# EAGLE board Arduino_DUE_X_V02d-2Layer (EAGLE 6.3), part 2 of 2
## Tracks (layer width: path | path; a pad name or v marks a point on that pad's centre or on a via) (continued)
PIN41  (via drill 0.41) (continued)
  Top 0.203: U1.67 39.49,19.79 39.62,19.91 53.24,19.91 54.15,20.83 55.68,20.83 56.49,20.02 58.12,20.02 v58.37,20.27 | v61.47,20.62 61.67,20.42 62.89,20.42 63.2,20.73 65.94,20.73 68.28,23.06 71.83,23.06 74.47,25.7 81.79,25.7 81.99,25.91 91.03,25.91 92.76,24.18 95.3,24.18 XIO.22
  Bottom 0.203: v58.37,20.27 58.73,20.62 v61.47,20.62
PIN42  (via drill 0.41)
  Top 0.203: v58.32,19.2 58.01,19.2 57.61,19.61 56.29,19.61 55.47,20.42 54.36,20.42 53.44,19.51 42.06,19.51 41.05,18.49 39.52,18.49 39.22,18.19 39.22,17.98 39.02,17.79 U1.71 | v61.47,19.61 61.87,20.02 63.09,20.02 63.4,20.32 66.14,20.32 68.38,22.55 71.93,22.55 74.68,25.3 82.09,25.3 82.3,25.5 90.83,25.5 93.17,23.16 93.67,23.16 XIO.23
  Bottom 0.203: v58.32,19.2 58.83,19.61 v61.47,19.61
PIN43  (via drill 0.41)
  Top 0.203: v39.93,17.78 39.42,17.27 38,17.27 U1.72 | v40.03,28.65 40.44,28.14 42.67,28.14 43.38,28.85 49.48,28.85 49.68,28.65 55.58,28.65 v55.68,28.75 | v57.4,41.35 58.32,42.27 60.55,42.27 61.37,43.08 62.08,43.08 63.7,41.45 65.84,41.45 66.04,41.25 75.39,41.25 76,41.86 79.65,41.86 80.06,42.27 82.09,42.27 82.6,42.77 84.94,42.77 v85.34,42.37 | XIO.24 97.74,24.08 97.74,33.83 97.23,34.34 90.73,34.34 90.53,34.54 89.31,34.54 89.1,34.34 87.88,34.34 86.56,35.66 86.56,36.68 v85.95,37.29
  Bottom 0.203: v39.93,17.78 39.93,18.19 43.18,21.44 43.18,27.03 42.06,28.14 41.15,28.14 40.64,28.65 v40.03,28.65 | v57.4,41.35 57.1,41.05 57.1,36.37 59.64,33.83 59.64,30.38 58.42,29.16 56.08,29.16 v55.68,28.75 | v85.34,42.37 85.45,42.27 85.45,41.25 85.14,40.95 85.14,38.1 v85.95,37.29
PIN44  (via drill 0.41)
  Top 0.203: U1.101 54.15,16.05 54.46,16.36 54.46,17.27 53.34,18.39 v52.83,18.39 | v63.4,16.66 63.7,16.36 69.29,16.36 75.59,10.06 85.55,10.06 89.41,13.92 89.41,16.76 92.96,20.32 XIO.25
  Bottom 0.203: v52.83,18.39 53.24,18.39 54.46,17.17 54.46,16.36 54.15,16.05 54.15,13.51 55.68,11.99 57.91,11.99 58.93,13.01 60.76,13.01 61.77,14.02 61.77,15.75 62.69,16.66 v63.4,16.66
PIN45  (via drill 0.41)
  Top 0.203: v53.75,16.76 53.75,16.26 53.65,16.15 U1.100 | XIO.26 95.3,19.1 92.86,19.1 89.92,16.15 89.92,13.72 85.85,9.65 75.39,9.65 69.09,15.95 62.18,15.95 59.33,13.11 v59.33,12.19
  Bottom 0.203: v59.33,12.19 58.62,11.48 55.58,11.48 53.75,13.31 v53.75,16.76
PIN46  (via drill 0.41)
  Top 0.203: U1.99 53.15,16.05 53.03,16.15 53.03,17.12 v51.77,18.39 | v62.59,15.24 62.89,15.54 68.89,15.54 75.18,9.25 86.06,9.25 90.42,13.61 90.42,15.44 92.76,17.78 XIO.27
  Bottom 0.203: v51.77,18.39 53.03,17.12 53.03,15.85 53.34,15.54 53.34,13.11 55.47,10.97 59.64,10.97 62.59,13.92 v62.59,15.24
PIN47  (via drill 0.41)
  Top 0.203: v52.22,16.87 52.63,16.46 52.63,15.24 U1.98 | XIO.28 95.2,16.46 93.37,16.46 90.93,14.02 90.93,13.41 84.84,7.32 79.86,7.32 78.33,8.84 74.98,8.84 68.68,15.14 64.52,15.14 v64.21,14.83
  Bottom 0.203: v52.22,16.87 52.22,15.95 52.93,15.24 52.93,12.9 55.37,10.46 59.84,10.46 v64.21,14.83
PIN48  (via drill 0.41)
  Top 0.203: XIO.29 93.37,15.24 85.04,6.91 79.65,6.91 78.13,8.43 74.78,8.43 68.78,14.43 v65.23,14.43 | v50.7,18.39 51.51,17.58 51.51,16.56 52.15,15.93 U1.97
  Bottom 0.203: v50.7,18.39 51.51,17.58 51.51,15.95 52.53,14.94 52.53,12.7 55.27,9.96 60.76,9.96 v65.23,14.43
PIN49  (via drill 0.41)
  Top 0.203: XIO.30 95.3,14.02 92.76,14.02 85.24,6.5 79.45,6.5 77.93,8.03 74.57,8.03 68.89,13.72 61.98,13.72 58.83,10.57 53.65,10.57 v52.93,11.28 | v51.82,13.61 51.61,13.82 51.61,15.04 U1.96
  Bottom 0.203: v51.82,13.61 51.82,12.39 v52.93,11.28
PIN50  (via drill 0.41)
  Top 0.203: U1.95 51.13,16.13 51.04,16.22 51.04,16.73 v50.8,16.97 | v51.92,11.28 53.03,10.16 59.03,10.16 62.18,13.31 68.68,13.31 74.37,7.62 77.72,7.62 79.25,6.1 85.45,6.1 91.24,11.89 92.05,11.89 92.86,12.7 XIO.31
  Bottom 0.203: v50.8,16.97 50.8,16.46 51.1,16.15 51.1,12.09 v51.92,11.28
PIN51  (via drill 0.41)
  Top 0.203: XIO.32 95.3,11.48 91.44,11.48 85.65,5.69 79.05,5.69 77.52,7.21 74.17,7.21 68.48,12.9 62.38,12.9 59.23,9.75 52.43,9.75 v51.92,10.26 | 50.6,15.23 U1.94 50.65,16 50.09,16.56 50.09,17.88 v49.58,18.39
  Bottom 0.203: v49.58,18.39 50.09,17.88 50.09,15.85 50.7,15.24 50.7,11.48 v51.92,10.26
PWM2  (via drill 0.41)
  Top 0.203: U1.144 59.54,34.75 60.86,34.75 v61.06,34.54
  Bottom 0.203: v61.06,34.54 60.15,34.54 57.91,36.78 57.91,39.62 58.83,40.54 58.83,48.97 58.42,49.38 PWML.3 58.42,50.9
PWM3  (via drill 0.41)
  Top 0.203: v56.49,31.8 56.69,32 58.32,32 58.62,32.31 59.54,32.31 U1.139
  Bottom 0.203: PWML.4 55.88,49.38 55.58,49.07 55.58,48.06 55.88,47.75 55.88,36.68 55.58,36.37 55.58,33.43 56.49,32.51 v56.49,31.8
PWM5  (via drill 0.41)
  Top 0.203: U1.136 58.62,30.79 58.22,31.19 57.51,31.19 57,30.68 54.76,30.68 54.46,30.38 51.41,30.38 v51.1,30.68
  Bottom 0.203: v51.1,30.68 51.1,34.85 51.61,35.36 51.61,37.39 52.22,37.9 52.22,38.71 53.14,39.62 53.14,46.43 50.8,48.77 PWML.6
PWM6  (via drill 0.41)
  Top 0.203: v57.81,30.48 58.32,30.48 58.52,30.28 59.54,30.28 U1.135 | PWML.7 48.26,49.51 48.59,49.17 55.88,49.17 v56.39,48.67
  Bottom 0.203: v57.81,30.48 57.81,31.9 55.98,33.73 55.98,35.66 56.29,35.97 56.29,48.56 v56.39,48.67
PWM7  (via drill 0.41)
  Top 0.203: U1.134 59.66,29.79 59.64,29.77 57.51,29.77 57,30.28 54.97,30.28 54.66,29.97 50.49,29.97 50.39,30.07 45.41,30.07 v45.11,30.38
  Bottom 0.203: v45.11,30.38 45.11,33.53 44.6,34.04 44.6,37.59 44.5,37.69 44.5,38.51 44.81,38.81 44.81,45.41 45.11,45.72 45.11,48.16 45.72,48.77 PWML.8
PWM8  (via drill 0.41)
  Top 0.203: v42.57,29.77 42.67,29.67 50.09,29.67 50.29,29.46 54.76,29.46 55.17,29.87 56.79,29.87 57.4,29.26 59.54,29.26 U1.133
  Bottom 0.203: PWMH.1 41.66,48.77 40.84,47.95 40.84,38.41 41.76,37.49 41.76,34.75 42.47,34.04 42.47,29.87 v42.57,29.77
PWM9  (via drill 0.41)
  Top 0.203: U1.132 59.43,28.79 59.33,28.78 57.28,28.78 56.59,29.46 55.37,29.46 54.97,29.06 49.99,29.06 49.78,29.26 43.18,29.26 42.77,28.85 v41.45,28.85
  Bottom 0.203: PWMH.2 39.12,49.07 40.44,47.75 40.44,38.2 40.95,37.69 40.95,34.34 42.06,33.22 42.06,30.28 41.45,29.67 v41.45,28.85
PWM11  (via drill 0.41)
  Top 0.203: v48.06,38.51 48.06,37.9 48.16,37.8 48.16,36.98 U1.20 | v39.32,45.52 39.73,45.52 39.83,45.41 44.7,45.41 45.31,46.02 46.43,46.02 46.74,46.33 47.55,46.33 47.95,45.92 47.95,45.41 v48.46,44.91
  Bottom 0.203: v48.46,44.91 47.85,44.3 47.85,39.22 48.06,39.01 v48.06,38.51 | PWMH.4 34.04,49.07 35.15,47.95 37.19,47.95 39.32,45.82 v39.32,45.52
PWM12  (via drill 0.41)
  Top 0.203: U1.21 47.65,35.46 v47.95,35.15 | v47.24,49.28 44.2,49.28 43.99,49.48 42.47,49.48 42.27,49.28 31.8,49.28 31.5,49.58 PWMH.5
  Bottom 0.203: v47.95,35.15 47.75,35.36 47.75,37.69 47.35,38.1 47.35,39.01 47.45,39.12 47.45,44.91 48.36,45.82 48.36,48.16 v47.24,49.28
PWM13  (via drill 0.41)
  Top 0.203: 21.34,28.25 IC1.3 | U1.68 35.87,19.3 35.78,19.29 31.27,19.29 v30.79,18.8
  Top 0.305: v22.96,28.25 21.34,28.25
  Bottom 0.203: PWMH.6 26.92,48.77 26.92,34.19 22.96,30.23 v22.96,28.25 23.47,28.25 27.33,24.38 27.43,24.38 28.75,23.06 28.75,20.83 v30.79,18.8
RD+
  Top 0.254: IC6.29 17.94,23.41 16.26,25.09 R20.1
RD-
  Top 0.254: IC6.30 17.44,23 16.46,23.98 15.04,23.98 14.98,24.02 R19.1
RESET2  (via drill 0.41)
  Top 0.254: ICSP1.5 26.01,17.27 26.01,18.29 26.21,18.49 26.21,19.33 D2.A | R13.1 22.55,23.84 v22.55,22.45 21.95,22.45 21.54,22.05 21.54,21.54 21.26,21.26 IC6.24
  Bottom 0.254: v22.55,22.45 23.37,23.27 24.38,23.27 24.89,22.76 24.89,20.73 24.49,20.32 24.49,18.85 25.91,17.37 | 25.96,17.32 ICSP1.5
  Bottom 0.305: 25.91,17.37 25.96,17.32
RESET_CMD
  Top 0.254: IC6.22 21.97,20.26 R23.1
RX  (via drill 0.41)
  Top 0.203: U1.27 44.65,35.01 45.31,34.34 v48.67,34.34 | v49.07,47.85 49.58,48.36 52.02,48.36 52.73,47.65 53.14,47.65 54.05,48.56 55.47,48.56 56.08,47.95 57.71,47.95 58.52,48.77 62.99,48.77 63.5,49.28 PWML.1 63.5,52 62.92,52.58 18.64,52.58 17.68,51.61 17.68,48.46 17.41,48.2 12.58,48.2 v12.2,48.58
  Top 0.254: IC10.4 13.95,15.45 v13.38,16.4
  Bottom 0.203: v48.67,34.34 48.67,35.76 48.77,35.87 48.77,38.91 48.26,39.42 48.26,43.69 49.28,44.7 49.28,46.13 49.07,46.33 v49.07,47.85 | v13.38,16.4 13.38,16.83 14.22,17.68 14.22,20.02 16.15,21.95 16.15,23.67 13.11,26.72 13.11,40.95 13.82,41.66 13.82,43.89 13.11,44.6 13.11,47.04 12.19,47.95 v12.19,48.57 v12.2,48.58
RXD0  (via drill 0.41)
  Top 0.203: COMMUNICATION.2 71.12,49.07 70.81,48.77 69.39,48.77 67.97,47.35 65.13,47.35 64.52,47.95 58.93,47.95 58.12,47.14 55.68,47.14 55.07,47.75 54.46,47.75 53.54,46.84 52.32,46.84 51.82,47.35 50.8,47.35 v50.09,46.63 | U1.18 49.15,37.62 49.48,37.95 v49.48,38.41
  Bottom 0.203: v50.09,46.63 50.09,45.52 49.78,45.21 49.78,44.6 48.67,43.48 48.67,39.62 49.48,38.81 v49.48,38.41
RXD1  (via drill 0.41)
  Top 0.203: v58.83,38.71 56.07,38.71 55.68,38.32 55.68,36.98 U1.5 | COMMUNICATION.4 76.2,48.36 75.79,47.95 70.92,47.95 v70.61,47.65
  Bottom 0.203: v58.83,38.71 58.83,39.93 59.23,40.34 59.23,47.14 60.25,48.16 70.1,48.16 v70.61,47.65
RXD2  (via drill 0.41)
  Top 0.203: U1.3 56.65,37.75 56.79,37.9 57.81,37.9 58.12,37.59 59.44,37.59 60.25,38.41 v60.66,38.41 | COMMUNICATION.6 81.28,48.46 80.87,48.06 79.96,48.06 79.45,47.55 77.42,47.55 77.01,47.14 72.95,47.14 v72.64,46.84
  Bottom 0.203: v60.66,38.41 61.37,39.12 61.37,39.83 60.45,40.74 60.45,46.53 60.86,46.94 66.34,46.94 67.16,46.13 71.93,46.13 v72.64,46.84
RXL  (via drill 0.41)
  Top 0.203: 55.17,15.23 U1.103 55.15,14.1 v54.86,13.92 | v32.31,15.75 33.73,15.75 34.54,16.56 35.26,16.56 35.56,16.26 40.34,16.26 41.45,17.37 43.38,17.37 44.4,18.39 v44.91,18.39
  Top 0.508: RX.C 7.92,33.33 6.81,32.21 v6.81,29.77
  Bottom 0.203: v54.86,13.92 54.86,17.37 53.14,19.1 48.06,19.1 47.75,18.8 47.75,17.88 47.24,17.37 45.92,17.37 v44.91,18.39 | v32.31,15.75 29.67,13.11 29.67,11.89 28.65,10.87 23.77,10.87 22.15,9.25 17.17,9.25 14.02,12.39 5.89,12.39 3.56,14.73 3.56,16.97 6.81,20.22 v6.81,29.77
RXL-U2
  Top 0.254: IC6.10 16.94,16.24 15.7,15 15.7,13.6 15,12.9 15,12.87 14.33,12.19 7.62,12.19 6.6,13.21 6.6,14.02 5.38,15.24 5.38,16.49 RX1.C
SCK2  (via drill 0.41)
  Top 0.254: IC6.15 19.44,16.08 v18.9,15.54
  Bottom 0.203: v18.9,15.54 18.9,16.87 19.61,17.58 21.13,17.58 22.76,15.95 24.74,15.95 ICSP1.3
SCL0-3  (via drill 0.41)
  Top 0.203: v57.71,28.04 57.25,27.64 54.76,27.64 54.56,27.84 47.09,27.84 v46.99,27.74 | v46.99,18.39 46.99,17.42 46.84,17.27 46.84,16.46 47.14,16.15 U1.87 | v85.95,38.41 85.34,39.01 81.48,39.01 81.42,38.95 80.5,38.95 79.5,37.95 | 79.5,37.95 78.23,36.68 68.89,36.68 67.16,38.41 64.92,38.41 63.09,36.58 63.09,35.36 62.48,34.75 v62.48,33.43 | RN5.7 80.77,36.68 79.5,37.95
  Bottom 0.203: v62.48,33.43 62.08,33.43 61.37,32.72 61.09,32.72 60.55,32.18 60.55,30.07 58.52,28.04 v57.71,28.04 | v46.99,18.39 46.94,24.23 46.63,24.54 46.63,27.38 v46.99,27.74
  Bottom 0.254: COMMUNICATION.8 86.26,50.7 86.26,42.16 85.95,41.86 v85.95,38.41
SCL1  (via drill 0.41)
  Top 0.203: 38,18.29 U1.70 37.19,18.29 37.08,18.39 34.95,18.39 34.34,17.78 33.63,17.78 33.53,17.88 v32.41,17.88 | PWMH.10 18.8,50.29 19.71,49.38 22.55,49.38 23.27,48.67 26.31,48.67 27.03,49.38 29.77,49.38 v29.87,49.48
  Bottom 0.203: v29.87,49.48 29.87,46.94 29.46,46.53 29.46,42.06 28.85,41.45 28.85,32.26 29.87,31.24 29.87,24.89 31.8,22.96 31.8,20.32 32.31,19.81 32.31,17.98 v32.41,17.88
SDA0-3  (via drill 0.41)
  Top 0.203: U1.86 46.63,15.34 | 46.63,15.34 46.69,15.24 | 46.63,15.34 46.63,16.01 46.38,16.26 46.38,17.98 v45.97,18.39 | v55.58,23.98 55.37,23.67 52.73,23.67 51.82,22.76 46.63,22.76 46.33,23.06 v45.97,23.06 | v79.45,36.47 79.25,36.47 78.94,36.17 71.22,36.17 v69.6,34.54
  Top 0.254: RN5.8 80.04,35.88 v79.45,36.47
  Bottom 0.203: v45.97,18.39 v45.97,23.06 | v55.58,23.98 55.68,25.2 57.3,26.82 58.52,26.82 61.77,30.07 61.77,31.29 62.79,32.31 66.95,32.31 69.09,34.54 v69.6,34.54
  Bottom 0.254: COMMUNICATION.7 83.82,43.69 82.91,42.77 82.91,40.44 82.7,40.23 82.7,38.2 81.99,37.49 80.47,37.49 v79.45,36.47
SDA1  (via drill 0.41)
  Top 0.203: v52.93,48.46 52.63,48.77 48.77,48.77 48.56,48.56 46.94,48.56 46.63,48.87 44.4,48.87 43.38,47.85 43.08,47.85 42.47,48.46 38.51,48.46 38,47.95 28.75,47.95 28.55,48.16 27.74,48.16 27.03,47.45 20.83,47.45 v20.02,48.26 | U1.9 53.65,36.78 53.65,35.56 v52.83,34.75
  Bottom 0.203: v52.93,48.46 53.54,47.85 53.54,39.42 52.63,38.51 52.63,35.56 52.83,35.36 v52.83,34.75 | v20.02,48.26 20.02,48.97 21.03,49.99 21.03,50.6 21.13,50.7 PWMH.9
SPCK  (via drill 0.41)
  Top 0.203: v72.54,28.85 69.7,28.85 69.19,28.35 67.67,28.35 66.75,29.26 65.33,29.26 64.72,28.65 64.41,28.65 SPI.3 | U1.110 60.66,17.79 62.48,19.61 63.3,19.61 63.6,19.91 66.34,19.91 68.48,22.05 71.53,22.05 v71.73,21.84
  Bottom 0.203: v71.73,21.84 71.73,25.6 72.54,26.52 v72.54,28.85
SS0/PWM10  (via drill 0.41)
  Top 0.203: U1.102 54.66,15.24 54.66,15.95 54.86,16.15 54.86,17.48 53.65,18.69 53.65,19.1 | U1.111 59.54,18.29 59.03,18.29 58.73,17.98 57.35,17.98 57.15,18.19 56.13,18.19 55.78,18.54 55.78,19.51 55.27,20.02 54.56,20.02 53.65,19.1 | v46.33,48.16 44.3,48.16 43.59,47.45 42.88,47.45 42.27,48.06 41.45,48.06 40.95,47.55 39.01,47.55 v38.91,47.75 | 53.65,19.1 43.69,19.1 v43.38,18.8
  Bottom 0.203: v38.91,47.75 36.58,50.09 PWMH.3 | v46.33,48.16 46.74,47.75 46.74,46.94 45.92,46.13 45.92,45.31 45.62,45.01 45.62,38.81 45.92,38.51 45.92,37.8 45.01,36.98 45.01,34.44 45.82,33.63 45.82,29.67 44.81,28.65 44.81,20.22 v43.38,18.8
SS1/PWM4  (via drill 0.41)
  Top 0.203: v53.54,31.09 56.79,31.09 57.3,31.6 58.42,31.6 58.73,31.29 59.54,31.29 U1.137 | U1.112 58.96,18.79 58.65,18.49 57.61,18.49 57.1,18.9 v56.49,18.9
  Bottom 0.203: PWML.5 53.44,50.8 53.44,49.38 55.47,47.35 55.47,36.98 55.17,36.68 55.17,34.44 53.54,32.82 v53.54,31.09 53.54,22.35 56.49,19.41 v56.49,18.9
SW
  Top 0.406: 82.98,17.92 D4.P$1 | IC2.6 83.24,15.89 C42.2
  Top 0.61: C42.2 82.98,17.92
  Top 1.27: 82.21,20.79 L4.P$1
  Top 1.676: D4.P$1 82.21,20.79
  pour Top (isolate 0.406, no thermals): 85.55,24.28 82.8,24.28 80.57,22.15 80.57,17.48 80.98,17.17 81.69,17.17 82.09,16.76 82.09,14.43 83.52,14.43 83.52,20.32 85.55,22.35
TX  (via drill 0.41)
  Top 0.203: U1.2 57.15,36.02 56.69,35.55 56.69,35.11 v56.69,35.05 | v57.4,48.67 57.91,49.17 60.66,49.17 60.96,49.48 PWML.2
  Top 0.254: IC6.8 14.93,17.76 14.72,17.57 v14.73,16.85
  Bottom 0.203: v56.69,35.05 56.69,47.95 v57.4,48.67 | PWML.2 59.18,52.58 21.18,52.58 20.12,51.51 20.12,49.78 19.2,48.87 17.98,48.87 16.66,47.55 14.43,47.55 13.51,46.63 13.51,45.01 14.22,44.3 14.22,41.15 13.61,40.54 13.61,26.82 16.56,23.88 16.56,21.74 14.63,19.81 14.63,16.95 v14.73,16.85
TXD0  (via drill 0.41)
  Top 0.203: U1.17 49.65,35.39 v49.38,35.15 | v50.09,47.65 50.39,47.95 51.82,47.95 52.53,47.24 53.34,47.24 54.25,48.16 55.27,48.16 55.88,47.55 57.91,47.55 58.73,48.36 64.72,48.36 65.33,47.75 67.77,47.75 68.58,48.56 COMMUNICATION.1
  Bottom 0.203: v49.38,35.15 50.19,35.97 50.19,38.71 49.07,39.83 49.07,43.28 50.19,44.4 50.19,44.81 50.8,45.41 50.8,47.35 50.49,47.65 v50.09,47.65
TXD1  (via drill 0.41)
  Top 0.203: v54.46,35.05 55.12,35.61 55.12,36.83 55.12,36.84 U1.6 | COMMUNICATION.3 73.66,48.77 73.25,48.36 69.6,48.36 68.17,46.94 64.92,46.94 64.31,47.55 59.13,47.55 58.32,46.74 55.07,46.74 v54.76,47.04
  Bottom 0.203: v54.46,35.05 54.46,37.08 55.07,37.69 55.07,46.74 v54.76,47.04
TXD2  (via drill 0.41)
  Top 0.203: U1.4 56.15,38.06 56.39,38.3 58.01,38.3 58.32,38 59.23,38 v60.66,39.42 | COMMUNICATION.5 78.74,48.36 78.33,47.95 77.22,47.95 76.81,47.55 71.93,47.55 v71.63,47.24
  Bottom 0.203: v60.66,39.42 60.05,40.03 60.05,46.74 60.66,47.35 66.55,47.35 67.36,46.53 70.92,46.53 v71.63,47.24
TXL  (via drill 0.41)
  Top 0.203: v29.16,8.53 30.18,7.52 32,7.52 32.41,7.92 45.01,7.92 45.31,8.23 45.31,9.2 45.67,9.55 47.45,9.55 47.7,9.8 49.23,9.8 51.51,12.09 53.24,12.09 54.36,10.97 58.01,10.97 58.52,11.58 58.52,13.72 58.06,14.17 57.56,14.17 57.15,14.59 U1.107
  Top 0.508: TX.C 8.79,31.45 v8.03,30.68
  Bottom 0.203: v8.03,30.68 6.6,30.68 6.1,30.18 6.1,20.12 3.05,17.07 3.05,14.33 5.49,11.89 13.92,11.89 17.07,8.74 24.69,8.74 24.89,8.94 26.31,8.94 26.72,8.53 v29.16,8.53
TXL-U2
  Top 0.254: IC6.11 17.44,16.04 16.2,14.8 16.2,13.3 14.58,11.68 7.15,11.68 TX1.C
UOTGID  (via drill 0.41)
  Top 0.203: 48.11,26.57 48.46,26.92 54.25,26.92 54.46,26.72 58.01,26.72 58.58,27.29 U1.129
  Top 0.254: 48.11,26.57 43.43,26.57 42.72,27.28 41.1,27.28 40.64,26.82 v40.54,26.82 | v36.68,45.11 35.97,45.82 31.6,45.82 31.39,45.62 30.07,45.62 29.92,45.77 22.45,45.77 21.29,44.6 20.02,44.6 19.3,45.31 7.32,45.31 6.91,44.91 v5.79,44.91 | 4.06,37.44 4.37,37.44 | 4.37,37.44 5.36,37.44 v6.5,36.27 | USB1.4 4.39,37.45 arc45 4.37,37.44
  Top 0.305: Z5.2 5.67,44.79 v5.79,44.91
  Bottom 0.254: v40.54,26.82 39.52,26.82 37.59,28.75 37.59,34.54 36.78,35.36 36.78,45.01 v36.68,45.11 | v6.5,36.27 6.5,44.2 v5.79,44.91
UOTGVBOF  (via drill 0.41)
  Top 0.203: U1.128 59.49,26.77 58.78,26.77 58.32,26.31 54.15,26.31 54.05,26.42 48.67,26.42 48.36,26.11 42.77,26.11 v42.37,26.52 | v36.68,17.68 34.95,17.68 34.65,17.37 33.63,17.37 v33.33,17.07
  Top 0.305: v30.58,25.2 30.38,25.4 R3.1
  Bottom 0.203: v42.37,26.52 42.77,26.11 42.77,21.84 38.61,17.68 v36.68,17.68 | v33.33,17.07 33.33,17.68 33.12,17.88 33.12,19.71 32.31,20.52 32.31,23.47 v30.58,25.2
USBVCC  (via drill 0.41, 0.61)
  Top 0.305: R21.2 21.17,24.63 v21.84,25.3 | R2.2 19.16,43.12 18.57,43.61 C27.+
  Top 0.406: 13.71,43.8 C35.+
  Top 0.762: v15.34,28.25 14.83,28.25 14.63,28.45 14.38,28.45 T1.1
  Top 0.813: F1.1 14.63,41 14.63,43.79 | 14.63,43.79 14.43,43.79 14.04,43.8 C35.+ | 14.63,43.79 16.97,43.79 C27.+ | C27.+ 16.87,43.71 | C27.+ v16.97,41.66
  Bottom 0.406: v21.84,25.3 21.84,25.5 20.73,26.62 15.95,26.62 15.44,27.13 v15.34,28.25
  Bottom 0.813: v16.97,41.66 16.97,29.16 16.05,28.25 v15.34,28.25
USBVCCU2  (via drill 0.61)
  Top 0.254: IC6.31 16.94,22.59 16.46,23.06
  Top 0.305: 16.46,23.06 11.99,23.06 11.79,23.27 T2.1 | C28.1 3.5,31.05 F2.1
  Top 0.61: T2.1 10.74,23.88 10.74,24.21 v10.67,24.28 | v6.81,33.83 6.28,33.83 F2.1
  Bottom 0.61: v10.67,24.28 10.46,24.28 9.45,25.3 9.45,28.65 10.06,29.26 10.06,32 8.94,33.12 7.52,33.12 v6.81,33.83
VBG  (via drill 0.41)
  Top 0.203: v39.42,33.12 39.24,33.3 38.23,33.3 U1.40 | v38.41,37.54 35.92,37.54 35.51,37.13 31.45,37.13 31.29,37.29 29.55,37.29 C25.1 29.26,37.27 29.26,37.8 29.06,38 28.04,38 27.84,37.8 26.72,37.8 26.49,37.57 R7.2
  Bottom 0.203: v38.41,37.54 38.41,36.88 39.42,35.87 v39.42,33.12
VDDANA  (via drill 0.41)
  Top 0.203: 40.12,15.01 U1.73
  Top 0.305: v39.42,15.01 40.12,15.01
  Top 0.406: v39.42,15.01 39.05,15.38 C10.2 35.6,15.38 35.15,14.94 34.75,14.94 33.83,14.02 L1.2
  Top 0.508: C3.+ v39.42,9.55
  Bottom 0.406: v39.42,15.01 v39.42,9.55
VDDOUT  (via drill 0.41, 0.61)
  Top 0.203: 38,22.78 U1.61 38.2,22.76 | 35.36,30.48 C14.2 | 59.54,24.79 U1.124 | 35.36,25.4 C15.2 | 54.8,12.9 C16.2 | 36.37,43.79 L5.1 | C17.2 61.57,23.77 | 32.72,21.54 32.92,21.74 | C11.+ 32.56,22.3 32.51,22.35
  Top 0.254: 59.54,24.79 58.73,24.79 58.57,24.64 57.35,24.64 57.2,24.69 57.15,24.79 | C12.2 34.28,21.68 34.95,21.74 | U1.124 60.8,24.79 C17.2
  Top 0.279: U1.45 36.68,30.79 | U1.10 53.15,37.91 v53.44,38.2 | 55.32,16.56 55.65,16.29 U1.104 55.65,13.48 55.07,12.9 C16.2 | 35.46,25.3 35.46,25.4 C15.2 | 38,22.78 36.6,22.78 36.68,22.76
  Top 0.292: 36.49,25.29 U1.56 39.36,25.29
  Top 0.305: 35.36,30.48 v36.37,30.48 36.68,30.79 | 36.49,25.29 v36.37,25.3 35.46,25.3 | C13.2 53.44,39.32 v53.44,38.2 | 39.36,25.29 39.93,25.86 | 55.32,16.56 55.32,18.85 v55.07,19.2
  Top 0.406: 57.15,24.79 53.95,24.79 53.34,24.18 52.43,24.18 51.82,23.57 v51.1,23.57 51.16,23.52 51.16,24.69 50.34,25.5 42.16,25.5 41.81,25.86 39.93,25.86 | 36.68,22.76 v35.66,21.74
  Top 0.61: v35.36,43.59 35.41,43.79 36.37,43.79 36.37,43.84
  Top 0.813: v35.66,21.74 34.95,21.74 34.75,21.95 33.53,21.95 33.33,21.74 32.92,21.74 32.51,21.74 32.51,22.35
  Bottom 0.406: v53.44,38.2 53.44,36.37 53.65,36.17 53.65,34.24 52.73,33.43 52.73,26.21 52.83,26.11 52.83,25.3 v51.1,23.57 52.02,23.57 53.03,22.55 53.03,22.05 55.07,20.02 v55.07,19.2
  Bottom 0.61: v36.37,30.48 36.37,31.09 33.83,33.63 33.83,39.12 35.36,40.64 v35.36,43.59
  Bottom 0.813: v36.37,30.48 v36.37,25.3 36.37,22.45 v35.66,21.74
VDDOUTMI  (via drill 0.41)
  Top 0.203: C2.+ 29.11,39.77 29.06,39.83 | 31.29,39.42 L2.2
  Top 0.254: 35.39,32.78 35.36,32.78 35.36,32.72 C9.2
  Top 0.279: U1.41 35.39,32.78
  Top 0.305: 35.39,32.78 35.36,32.82 v35.36,33.58
  Top 0.406: v34.85,38.15 32.56,38.15 31.29,39.42
  Top 0.61: L2.2 30.13,39.42 C2.+
  Bottom 0.406: v35.36,33.58 35.36,37.64 v34.85,38.15
VDDPLL
  Top 0.203: 41.96,42.67 42.27,43.08 | 42.27,43.69 42.27,43.28 42.27,43.08 | 42.27,43.08 C33.+ | L5.2 38.61,43.79
  Top 0.279: U1.34 41.15,39.52
  Top 0.406: 41.15,39.52 41.96,40.34 | 41.96,40.34 41.96,42.67 | C32.2 41.96,40.34
  Top 0.61: 38.61,43.79 39.83,43.79 40.13,43.48 42.06,43.48 42.27,43.28
VIN  (via drill 0.41, 0.61)
  Top 0.305: v27.84,29.16 26.92,30.07 RN4.6
  Top 0.406: 84.96,15.67 v84.73,15.54
  Top 0.61: 84.96,15.67 C41.+ 87.21,15.02 87.21,14.06 87.07,13.92 R10.1 | v84.73,15.54 v84.73,14.33 83.92,13.51 IC2.5
  Top 1.016: v32,6.6 32.41,6.6 32.72,6.91 45.21,6.91 45.52,6.6 v45.72,6.6 | v32,6.6 32.11,6.6 | v32,6.6 27.23,6.6 24.22,3.59 PC1.+ 21,3.59 D5.P$1
  Bottom 0.305: v27.84,29.16 27.84,28.45 28.65,27.64 28.65,23.88 29.26,23.27 29.26,21.54 31.6,19.2 31.6,17.58 33.22,15.95 33.22,7.62 32.61,7.01 v32,6.6
  Bottom 0.61: v84.73,14.33 82.6,14.33 77.72,9.45 73.97,9.45 68.89,4.37 50.39,4.37 49.07,3.05 49.07,2.34 48.46,1.73 46.53,1.73 POWER.8
  Bottom 1.016: POWER.8 v45.72,6.6
  pour Top (no thermals): 87.78,16.56 85.04,16.56 84.12,15.65 84.12,13.61 85.04,13.61 85.24,13.82 85.24,14.43 85.55,14.73 87.68,14.73 87.88,14.94 87.88,16.46
  pour Bottom: 84.12,16.15 85.55,16.15 85.55,13.72 84.12,13.72
VIN+
  Top 1.016: X2.2 11.71,8.33 13.82,8.33 15.53,6.62 L6.2
VUCAP
  Top 0.254: IC6.27 18.94,23.87 C38.1
XIN
  Top 0.203: 36.47,41.76 Y1.1 | 36.47,41.76 36.27,41.35 | 36.47,41.76 36.58,41.86 Y1.1 | U1.36 40.15,37.58 39.37,38.35 35.87,38.35 34.91,39.31 34.91,40.2 | C22.1 34.91,40.2 | 34.91,40.2 35.55,40.2 35.97,40.64 35.97,41.15 Y1.1
XIN32
  Top 0.203: U1.48 38,29.26 37.29,29.26 36.98,29.57 33.12,29.57 32.31,30.38 31.24,30.38 | C24.1 31.01,30.48 | 31.01,30.48 31.24,30.38 | 31.24,30.38 Y2.P$2 31.01,30.48
XOUT
  Top 0.203: 39.57,39.47 38.41,39.47 38.41,39.62 Y1.3 38.41,39.42 | 39.57,39.47 39.58,39.47 40.23,40.13 40.23,40.84 C21.1 | U1.35 40.64,36.98 40.64,37.85 39.98,38.51 39.57,38.91 39.57,39.47
XOUT32
  Top 0.203: U1.49 38,28.79 38,28.8 37.03,28.8 36.68,29.16 33.53,29.16 32.31,27.94 31.7,27.94 | C23.1 31.22,27.84 | 31.22,27.84 31.7,27.94 | 31.7,27.94 Y2.P$1 31.22,27.84
XT1
  Top 0.254: C39.1 R9.1 | Y4.1 8.62,15.03 9.55,15.95 9.55,17.48 9.14,17.88 9.14,18.45 R9.1 | IC6.1 12.82,21.26 11.68,20.12 11.07,20.12 10.36,19.41 9.35,19.41 9.11,19.16 R9.1
XT2
  Top 0.254: 10.06,18.55 R9.2 C40.1 | Y4.3 10.7,18.16 C40.1 | IC6.2 13.24,20.76 12.09,19.61 11.38,19.61 11.04,19.27 C40.1
XUSB  (via drill 0.41)
  Top 0.254: USB1.1 4.42,39.4 arc45 4.47,39.4 | U1.39 36.62,33.78 v36.58,33.73 | v35.15,44.91 35.05,44.91 34.75,45.11 29.67,45.11 29.46,45.31 22.66,45.31 21.13,43.79 19.91,43.79 18.9,44.81 11.89,44.81 11.07,43.99 C26.1
  Top 0.305: C26.1 11.01,41.71 F1.2
  Top 0.4: 5.84,39.4 4.47,39.4
  Top 0.406: 4.47,39.4 4.45,39.4 | 6.15,39.93 6.15,39.73 5.84,39.4
  Top 0.813: 6.15,39.93 6.15,41.6 7.72,43.18 8.74,43.18 10.06,41.86 10.06,40.82 F1.2
  Bottom 0.254: v36.58,33.73 36.47,33.73 36.27,33.93 36.27,44.09 35.46,44.91 v35.15,44.91
XVCC
  Top 0.406: J3.P1 4.85,23.55 5.38,24.08 5.38,27.92 F2.2

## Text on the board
tPlace: 9 | 8 | 7 | 6 | 5 | 4 | 3 | 2 | 1 | 0 | 22 | 14 | 15 | 16 | 17 | 18 | 19 | 20 | 21 | 13 | 12 | 11 | 10 | 24 | 26 | 28 | 30 | 31 | 32 | 33 | 34 | 35 | 36 | 37 | 38 | 39 | 40 | 41 | 42 | 43 | 44 | 45 | 46 | 47 | 48 | 49 | 50 | 51 | 52 | 53 | www.arduino.cc | 0 | 1 | 2 | 3 | 4 | 5 | 6 | 7 | 8 | 9 | 10 | 11 | DAC0 | DAC1 | CANRX | CANTX
tNames: M.Banzi | 5V | D.Cuartielles | T.Igoe | G.Martino | D.Mellis | GND | SCL1 | SDA1 | AREF | PWM | TX | RX | TX0 | RX0 | TX1 | RX1 | TX2 | RX3 | SDA | SCL | 1 | MADE IN | ITALY | DIGITAL | Arduino | DUE | ANALOG IN | GND | IOREF | RESET | 3V3 | 5V | GND | VIN
ReferenceLC: PC2 | PC1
